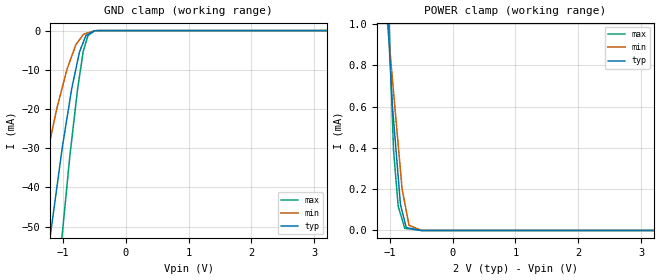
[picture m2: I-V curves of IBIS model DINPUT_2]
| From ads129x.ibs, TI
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|   DINPUT 2.0V Model
[Model]   DINPUT_2
Model_type   Input
|for ADS1299 products
|Signals   DIN, CLKSEL, START, _CS, _RESET, _PWDN, RESV1
Vinl = 0.4
Vinh = 1.6
|   typ   min   max
|   (nom PVT)   (Fast PVT)   (slow PVT)
|C_comp from LC tank measurement(L=1nH)
C_comp   1.762E-12   1.413E-12   2.080E-12
| Where   nom PVT is  Nominal Process, 2V, 27C
|   Fast PVT is Strong Process, 2.2V, -40C
|   Slow PVT is Weak Process, 1.8V, 85C
[Voltage Range]   2   1.8   2.2
[Temperature Range]   27   85   -40
[Power Clamp Reference]   2   1.8   2.2
[GND Clamp Reference]   0   0   0
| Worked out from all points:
|   GND clamp passes 1 mA (typ) near -0.60 V on its own axis
|   POWER clamp passes 1 mA (typ) near -1.02 V on its own axis
[GND Clamp]
|   Voltage   I(typ)   I(min)   I(max)
-2V       -165mA     -103.7mA   -225.8mA
-1.501V   -92.94mA   -52.98mA   -136.6mA
-1.42V    -81.21mA   -45.88mA   -122mA
-1.201V   -52.44mA   -27.8mA    -83.48mA
-1.004V   -29.36mA   -14.21mA   -51.08mA
-893.3mV  -18.24mA   -8.053mA   -32.73mA
-766.2mV  -7.786mA   -3.015mA   -14.98mA
-732.1mV  -5.289mA   -2.272mA   -11.33mA
-669.4mV  -2.756mA   -907.9uA   -4.968mA
-600.8mV  -975.6uA   -568.8uA   -1.286mA
-469.4mV  -26.5uA    -23.94uA   -30.72uA
3.994V    0A         0A         0A
[POWER Clamp]
|   Voltage   I(typ)   I(min)   I(max)
-2V       13.12mA    10.41mA    16.44mA
-1.035V   1.096mA    1.005mA    1.318mA
-1.011V   911.5uA    919.2uA    1.019mA
-1.005V   876.1uA    898.5uA    953.1uA
-960.4mV  615.3uA    745.1uA    568.7uA
-939.7mV  537.9uA    673.3uA    391.2uA
-867.1mV  267.1uA    422uA      122.3uA
-827.1mV  122.7uA    283.5uA    78.12uA
-760.4mV  42.06uA    132.4uA    10.33uA
-693.7mV  11.43uA    25.58uA    7.717uA
-494.6mV  0A         53.96nA    0A
3.994V    0A         0A         0A
